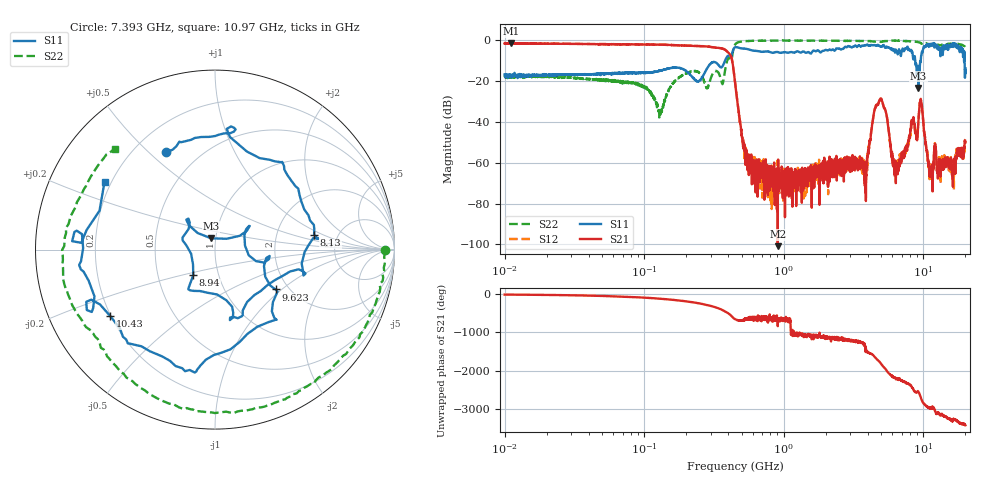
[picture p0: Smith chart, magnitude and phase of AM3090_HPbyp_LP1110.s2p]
# Hz S DB R 50
!freq MagS11 AngS11 MagS21 AngS21 MagS12 AngS12 MagS22 AngS22
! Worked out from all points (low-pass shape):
!   3201 points, 10 MHz to 20 GHz, reference 50 ohm
!   highest |S21| = -1.51 dB at 11.1 MHz (marker M1); lowest = -100.9 dB at 905.5 MHz (marker M2)
!   |S21| within 3 dB of the highest: start of sweep to 374.2 MHz
!   lowest |S11| = -23.5 dB at 9.22 GHz (marker M3), VSWR 1.14, Z = 47.5 + j6.01 ohm
!   |S11| at or under -10 dB: start of sweep to 380 MHz; 8.737 GHz to 9.576 GHz (839.1 MHz wide, 9.16 % of centre); 19.73 GHz to end of sweep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
!   |S22| runs from -37.9 to -0.2 dB; largest |S21 - S12| = 0.029
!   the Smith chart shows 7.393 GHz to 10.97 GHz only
!   S11 on the Smith chart (normalised r, x): 7.393 GHz: 0.33, +0.57; 8.13 GHz: 3.32, +0.78; 8.94 GHz: 0.76, -0.22; 9.623 GHz: 1.71, -0.91; 10.43 GHz: 0.20, -0.28; 10.97 GHz: 0.17, +0.27
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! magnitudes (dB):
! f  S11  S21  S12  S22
! 10 MHz  -16.8  -1.7  -1.7  -17.4
! 11.1 MHz  -17.7  -1.5  -1.8  -17.5
! 35.55 MHz  -16.9  -1.9  -1.9  -18.8
! 126.1 MHz  -15.3  -2.3  -2.2  -33.2
! 194.7 MHz  -14.6  -2.7  -2.7  -16.7
! 372.5 MHz  -11.4  -4.5  -4.4  -18.4
! 447.2 MHz  -3.5  -20.4  -20.5  -2.3
! 547.3 MHz  -4.4  -60.2  -60.1  -0.5
! 905.5 MHz  -5.9  -100.9  -62.3  -0.3
! 1.59 GHz  -6.1  -63.3  -63.7  -0.3
! 3.793 GHz  -2.5  -65.1  -64.8  -0.5
! 4.902 GHz  -3.1  -29.3  -28.9  -0.9
! 5.639 GHz  -3.7  -44.3  -44.2  -0.4
! 6.335 GHz  -4.8  -63.6  -60.5  -0.3
! 7.393 GHz  -4.3  -53.3  -54.9  -0.5
! 8.13 GHz  -5.1  -43.7  -44.7  -0.6
! 8.94 GHz  -14.6  -48.0  -48.5  -0.9
! 9.22 GHz  -23.5  -39.1  -39.2  -1.0
! 9.623 GHz  -7.9  -29.7  -29.7  -1.6
! 10.43 GHz  -3.2  -50.8  -51.9  -1.6
! 10.97 GHz  -2.8  -59.9  -62.3  -2.0
! 20 GHz  -13.7  -50.1  -48.5  -3.5
